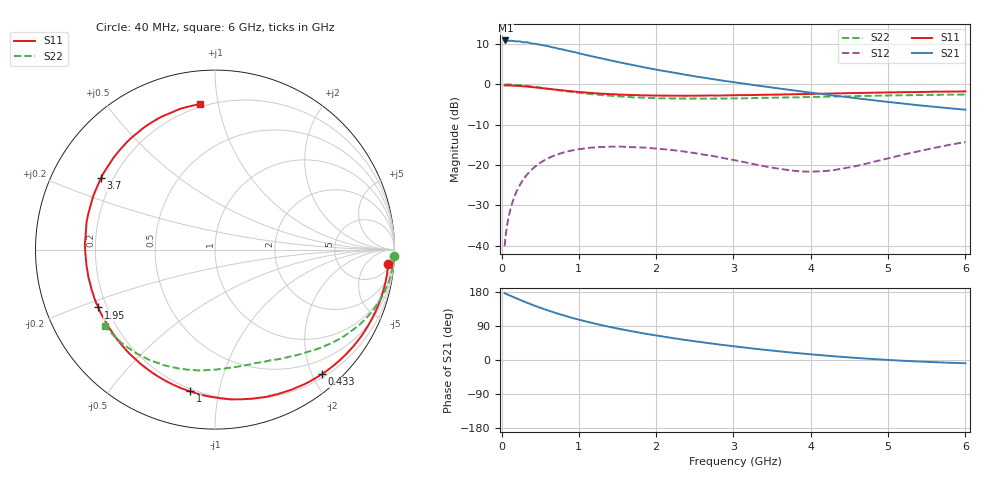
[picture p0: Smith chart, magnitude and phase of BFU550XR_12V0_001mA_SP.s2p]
! Filename:  P:\Prog\Test\Noise\ATS_data\Testdata_Net\03 Spar\BFU550XR_APG2013_45_C05_12p0V_001mA_SP_CM01_D.s2p
! Date/Time: Tue 06/Aug/2013 14:38:18
! BFU550XR_APG2013_45_C05_12p0V_1to35mA_SP_CM01_Bias1_R.s2p
! MDIF S-parameter v. bias file
! BFU550XR_APG2013_45_C05_12p0V_1to35mA_SP_CM01
! Date/time Fri Aug 02 14:58:10 2013
! bias mode 1
! bias variable = I_out
! VAR bias_var= 1
! VAR V_out= 12.0010
! VAR I_out= 0.9950
! VAR V_in= 0.7722
! VAR I_in= 0.0081
! Device data file deembeded for feedlines and parallel
! Original file: \03 Spar\BFU550XR_APG2013_45_C05_12p0V_001mA_SP_CM01_R.s2p
! Feed-files: PR006V01_02082013_Feed1.s2p, PR006V01_02082013_Feed2.s2p
! Parallel-file: PR006V01_02082013_Par.s2p
# MHz S MA R 50
!  Freq-MHz  S11-mag  S11-arg  S21-mag  S21-arg  S12-mag  S12-arg  S22-mag  S22-arg
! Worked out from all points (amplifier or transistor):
!   98 points, 40 MHz to 6 GHz, reference 50 ohm
!   highest |S21| = 10.9 dB at 50 MHz (marker M1)
!   |S21| within 3 dB of that: start of sweep to 965.3 MHz
!   unconditionally stable (mu >= 1): 3.441 GHz to 4.745 GHz
!   at 300 MHz: K = 0.08, MSG = 16.7 dB, |S12| = -23.1 dB
!   at 1.6 GHz: K = 0.38, MSG = 10.3 dB, |S12| = -15.5 dB
!   at 6 GHz: K = 0.77, MSG = 4.0 dB, |S12| = -14.3 dB
!   S11 on the Smith chart (normalised r, x): 40 MHz: 8, -21; 433 MHz: 0.25, -2.15; 1 GHz: 0.19, -0.82; 1.95 GHz: 0.17, -0.23; 3.7 GHz: 0.15, +0.28; 6 GHz: 0.18, +0.88
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40  0.9691 -4.8  3.479 176.4  0.009861 85.9  0.998 -2.1
50  0.9691 -5.9  3.489 175.0  0.01233 85.7  0.9983 -2.8
100  0.9664 -11.8  3.445 170.9  0.02454 82.0  0.9932 -5.9
180  0.9587 -21.2  3.405 163.8  0.04361 76.0  0.984 -10.6
240  0.9503 -28.2  3.393 158.6  0.05706 71.7  0.9736 -14.0
320  0.9365 -37.2  3.314 151.9  0.07395 66.1  0.9557 -18.4
433  0.915 -49.3  3.171 143.0  0.09527 58.7  0.9274 -23.9
600  0.8781 -66.3  2.974 130.8  0.1205 48.6  0.8803 -31.5
700  0.8571 -75.5  2.825 124.2  0.1325 43.2  0.8539 -35.6
850  0.828 -88.3  2.613 114.9  0.1468 36.1  0.8174 -40.8
1000  0.8021 -100.0  2.422 106.5  0.1568 29.6  0.7853 -45.6
1050  0.7953 -103.6  2.359 103.9  0.1588 27.6  0.7735 -47.1
1250  0.77 -117.0  2.133 94.0  0.1668 20.5  0.7434 -52.4
1500  0.7472 -131.7  1.892 83.1  0.1689 12.7  0.7107 -58.7
1950  0.7255 -153.7  1.55 66.4  0.1614 2.0  0.6766 -68.7
2050  0.7247 -157.9  1.488 63.2  0.1578 0.3  0.6707 -70.8
2500  0.7208 -175.3  1.256 49.3  0.1402 -6.5  0.6645 -79.9
3100  0.7334 165.0  1.029 33.9  0.1104 -7.6  0.6704 -91.7
3700  0.7496 147.9  0.8589 20.6  0.08673 3.6  0.6868 -103.3
4100  0.763 137.6  0.7667 13.2  0.08318 18.8  0.698 -110.9
5200  0.7981 112.1  0.5762 -2.1  0.1346 43.8  0.7296 -131.2
6000  0.8153 96.0  0.4842 -8.5  0.1923 42.1  0.7472 -145.4
